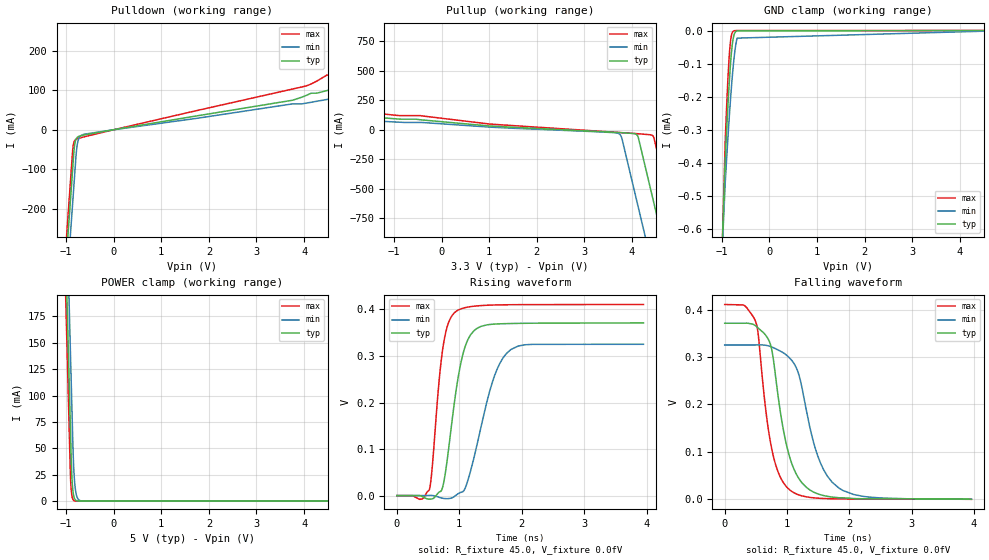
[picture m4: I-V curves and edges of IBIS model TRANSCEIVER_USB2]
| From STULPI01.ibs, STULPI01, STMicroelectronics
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[Model]   TRANSCEIVER_USB2
Model_type Output
Polarity   Non-Inverting
Enable   Active-Low
C_comp   4pF  NA  NA
Vmeas = 185mV
Cref  = 5.0pF
Rref  = 1.0MOhm
Vref  = 185mV
[Temperature Range] 25.0 125.0 -40.0
[Voltage Range] 3.3V 3.0V 3.6V
[POWER Clamp Reference] 5.0V 4.5V 5.5V
| variable   typ   min   max
[GND Clamp Reference] 0.0fV 0.0fV 0.0fV
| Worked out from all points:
|   slope of the pulldown table from 0 to 0.495 V, typ, clamps not added: 49.7 ohm
|   slope of the pullup table from 0 to 0.495 V, typ, clamps not added: 27.6 ohm
|   POWER clamp passes 1 mA (typ) near -0.80 V on its own axis
|   rising waveform, R_fixture 45.0, V_fixture 0.0fV: 20-80 % time 241ps typ, 368ps min, 171ps max; typ from 0 V to 0.371 V
|   falling waveform, R_fixture 45.0, V_fixture 0.0fV: 20-80 % time 301ps typ, 382ps min, 245ps max; typ from 0.371 V to 0 V
[POWER Clamp]
-5V       7.025A     7.098A     6.98A
-3.54V    4.543A     4.616A     4.498A
-910mV    71.87mA    144.5mA    27.03mA
-900mV    54.87mA    127.5mA    16.17mA
-880mV    25.35mA    93.53mA    5.785mA
-870mV    16.96mA    76.53mA    3.46mA
-850mV    7.596mA    44.07mA    1.238mA
-830mV    3.402mA    24.15mA    443.1uA
-810mV    1.524mA    13.24mA    158.6uA
-780mV    456.7uA    5.372mA    33.95uA
-660mV    3.689uA    145.6uA    71.42nA
5V        0A         0A         0A
[GND Clamp]
-5V       -17.5mA    -13.66mA   -21.39mA
-2.92V    -8.579mA   -6.769mA   -10.43mA
-930mV    -391.9uA   -460.3uA   -334.3uA
-880mV    -245.3uA   -339.5uA   -166.2uA
-840mV    -145.1uA   -251uA     -66.02uA
-820mV    -102.9uA   -210.1uA   -33.82uA
-800mV    -67.77uA   -171.9uA   -14.79uA
-780mV    -40.74uA   -136.7uA   -5.74uA
-750mV    -15.86uA   -90.74uA   -1.243uA
-710mV    -3.538uA   -44.76uA   -152.6nA
-680mV    -1.061uA   -22.92uA   -31.44nA
5V        10pA       9.012pA    9.5pA
[Pullup Reference] 3.3V 3.0V 3.6V
[Pulldown Reference] 0.0fV 0.0fV 0.0fV
[Pullup]
-3.3V     1.413A     1.784A     1.079A
-2.77V    512.5mA    883.5mA    195.5mA
-2.55V    151.1mA    509.4mA    186mA
-2.33V    134.1mA    135.4mA    178.9mA
-2.26V    132.6mA    93mA       176.1mA
3.71V     -23.8mA    -30.58mA   -22.83mA
3.79V     -25.54mA   -77.74mA   -24.93mA
4.12V     -54.25mA   -638.7mA   -33.82mA
4.36V     -453.6mA   -1.047A    -41.72mA
4.41V     -538.6mA   -1.132A    -45.16mA
4.47V     -640.6mA   -1.234A    -86.2mA
6.6V      -4.262A    -4.855A    -3.707A
[Pulldown]
-3.3V     -4.246A    -4.332A    -4.198A
-870mV    -115.1mA   -201mA     -67.43mA
-820mV    -38.81mA   -116mA     -27.95mA
-780mV    -21.67mA   -51.81mA   -23.83mA
-730mV    -16.72mA   -22.03mA   -21.73mA
5.21V     122.1mA    88.47mA    156.4mA
5.3V      124.9mA    106.6mA    160.1mA
5.55V     132.3mA    509.4mA    170.5mA
5.82V     139mA      968.5mA    181.5mA
6.09V     546.5mA    1.427A     192mA
6.34V     971.5mA    1.852A     195.1mA
6.6V      1.413A     2.294A     576.5mA
[Ramp]
dV/dt_r 222.65184mV/241.10317ps 195.08123mV/366.96565ps 246.36978mV/170.63002ps
dV/dt_f 222.58208mV/300.53042ps 194.91641mV/380.98856ps 246.32959mV/244.70531ps
R_load = 45.0
[Rising Waveform]
R_fixture   = 45.0
V_fixture   = 0.0fV
V_fixture_min = 0.0fV
V_fixture_max = 0.0fV
0s        7.031uV    11.19uV    5.22uV
522ps     -7.641mV   396.3uV    13.02mV
734ps     18.13mV    -5.66mV    313.3mV
814ps     83.55mV    -6.533mV   365.8mV
938ps     215.2mV    -268.3uV   394.6mV
1.054ns   301.3mV    8.12mV     402.4mV
1.178ns   344.8mV    51.31mV    405.9mV
1.526ns   368.2mV    241.9mV    409.4mV
1.826ns   369.7mV    313.8mV    410.1mV
3.95ns    371.1mV    325.1mV    410.6mV
|3.95000000E-09   3.71169237E-01  3.25316144E-01  4.10656483E-01
[Falling Waveform]
R_fixture   = 45.0
V_fixture   = 0.0fV
V_fixture_min = 0.0fV
V_fixture_max = 0.0fV
0s        371.2mV    325.3mV    410.7mV
300ps     371.2mV    325.3mV    409.8mV
500ps     365.3mV    325.3mV    373.4mV
712ps     334.1mV    323.1mV    138mV
844ps     230.7mV    315.6mV    62.44mV
1.044ns   88.62mV    297.5mV    20.01mV
1.192ns   43.65mV    262mV      9.318mV
1.5ns     11.37mV    89.31mV    2.505mV
1.836ns   3.373mV    23.59mV    944.4uV
3.96ns    199.1uV    455.5uV    107.2uV
